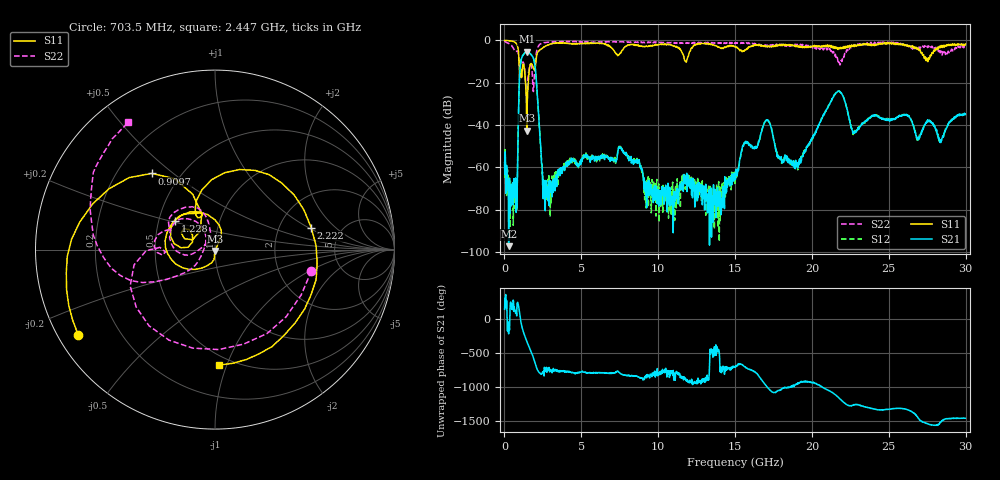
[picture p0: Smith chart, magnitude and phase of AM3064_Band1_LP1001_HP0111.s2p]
# Hz S DB R 50.0
!freq dBS11 angS11 dBS21 angS21 dBS12 angS12 dBS22 angS22
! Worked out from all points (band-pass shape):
!   1600 points, 10 MHz to 29.98 GHz, reference 50 ohm
!   highest |S21| = -5.34 dB at 1.453 GHz (marker M1); lowest = -97.3 dB at 272.4 MHz (marker M2)
!   |S21| within 3 dB of the highest: 1.118 GHz to 1.881 GHz (763 MHz wide, 50.9 % of centre)
!   lowest |S11| = -42.7 dB at 1.453 GHz (marker M3), VSWR 1.01, Z = 50.3 - j0.693 ohm
!   |S11| at or under -10 dB: 949.3 MHz to 2.043 GHz (1.094 GHz wide, 73.1 % of centre); 11.80199 GHz to 11.83974 GHz (37.75 MHz wide, 0.319 % of centre); 27.54048 GHz to 27.54524 GHz (4.759 MHz wide, 0.0173 % of centre)
!   |S22| runs from -25.6 to -0.3 dB; largest |S21 - S12| = 0.0076
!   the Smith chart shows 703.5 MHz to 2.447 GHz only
!   S11 on the Smith chart (normalised r, x): 703.5 MHz: 0.06, -0.29; 909.7 MHz: 0.35, +0.42; 1.228 GHz: 0.61, +0.21; 2.222 GHz: 3.04, +1.05; 2.447 GHz: 0.43, -0.94
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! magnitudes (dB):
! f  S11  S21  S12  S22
! 10 MHz  0.0  -57.7  -58.6  -0.3
! 272.4 MHz  -0.1  -97.3  -72.3  -1.5
! 703.5 MHz  -0.9  -74.4  -70.0  -5.2
! 909.7 MHz  -5.2  -35.9  -35.9  -6.8
! 1.228 GHz  -11.2  -6.8  -6.7  -10.4
! 1.453 GHz  -42.7  -5.3  -5.3  -24.8
! 1.922 GHz  -13.5  -9.4  -9.4  -19.0
! 2.222 GHz  -5.2  -35.1  -35.1  -2.6
! 2.447 GHz  -3.8  -58.6  -61.6  -1.3
! 2.859 GHz  -2.2  -66.6  -65.4  -0.9
! 5.015 GHz  -1.5  -57.5  -56.6  -0.7
! 7.564 GHz  -5.7  -50.7  -50.2  -0.6
! 10 GHz  -2.0  -70.9  -73.7  -1.0
! 15 GHz  -3.1  -64.3  -66.3  -1.4
! 17.05 GHz  -2.9  -37.7  -37.5  -2.7
! 18.04 GHz  -1.9  -56.9  -56.4  -1.9
! 19.99 GHz  -3.1  -46.3  -46.9  -3.1
! 21.7 GHz  -4.3  -24.1  -23.9  -10.4
! 22.75 GHz  -2.9  -43.6  -43.6  -2.0
! 25 GHz  -1.1  -37.9  -37.6  -1.0
! 28.35 GHz  -3.4  -46.9  -47.2  -5.8
! 29.98 GHz  -1.8  -34.9  -35.4  -3.1
